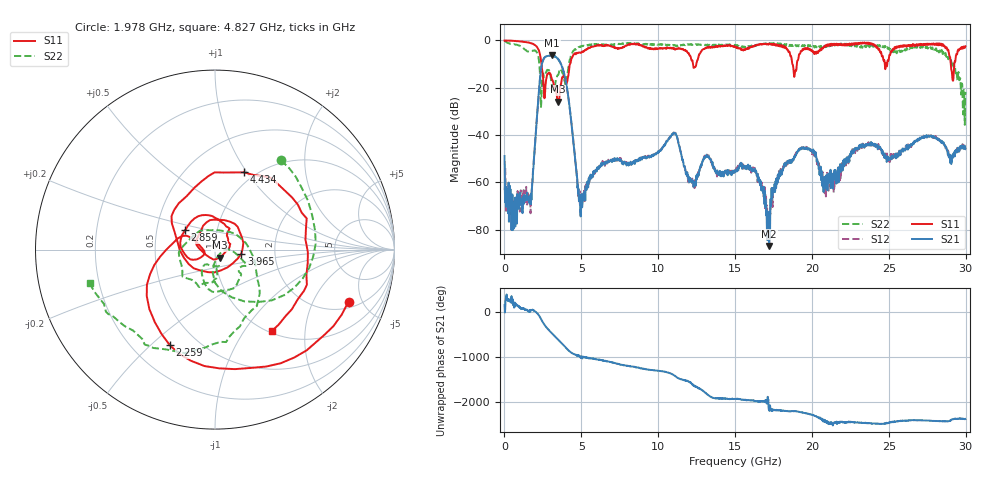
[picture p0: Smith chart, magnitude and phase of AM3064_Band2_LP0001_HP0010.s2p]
# Hz S DB R 50.0
!freq dBS11 angS11 dBS21 angS21 dBS12 angS12 dBS22 angS22
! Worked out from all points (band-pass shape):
!   1600 points, 10 MHz to 29.98 GHz, reference 50 ohm
!   highest |S21| = -6.29 dB at 3.103 GHz (marker M1); lowest = -86.9 dB at 17.22 GHz (marker M2)
!   |S21| within 3 dB of the highest: 2.465 GHz to 3.618 GHz (1.153 GHz wide, 37.9 % of centre)
!   lowest |S11| = -25.9 dB at 3.478 GHz (marker M3), VSWR 1.11, Z = 52.4 - j4.66 ohm
!   |S11| at or under -10 dB: 2.405 GHz to 4.263 GHz (1.858 GHz wide, 55.7 % of centre); 18.73 GHz to 19.02 GHz (291 MHz wide, 1.54 % of centre); 29.03 GHz to 29.26 GHz (229.6 MHz wide, 0.788 % of centre)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
!   |S22| runs from -35.7 to -0.2 dB; largest |S21 - S12| = 0.014
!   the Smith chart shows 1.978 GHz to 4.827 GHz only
!   S11 on the Smith chart (normalised r, x): 1.978 GHz: 2.42, -3.88; 2.259 GHz: 0.35, -0.58; 2.859 GHz: 0.70, +0.16; 3.965 GHz: 1.34, -0.06; 4.434 GHz: 0.89, +0.97; 4.827 GHz: 1.02, -1.35
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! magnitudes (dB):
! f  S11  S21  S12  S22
! 10 MHz  0.0  -48.9  -63.2  -0.2
! 553.6 MHz  -0.2  -68.8  -70.1  -1.6
! 1.603 GHz  -1.0  -67.3  -64.7  -4.7
! 1.978 GHz  -2.0  -44.6  -45.0  -4.2
! 2.259 GHz  -4.6  -19.9  -19.9  -9.6
! 2.859 GHz  -14.0  -6.5  -6.5  -12.6
! 3.103 GHz  -16.9  -6.3  -6.5  -19.3
! 3.478 GHz  -25.9  -7.8  -7.9  -14.6
! 3.965 GHz  -16.5  -16.5  -16.4  -19.1
! 4.434 GHz  -6.7  -39.6  -39.7  -5.0
! 4.827 GHz  -5.1  -65.3  -63.0  -2.8
! 5.015 GHz  -5.1  -65.0  -67.8  -2.6
! 10 GHz  -3.4  -47.5  -46.8  -1.7
! 15 GHz  -2.6  -55.8  -55.3  -1.9
! 16.32 GHz  -2.2  -55.7  -55.2  -2.0
! 17.22 GHz  -1.3  -86.9  -87.0  -1.5
! 17.99 GHz  -2.5  -55.4  -55.2  -1.4
! 19.99 GHz  -4.2  -46.7  -46.8  -2.0
! 20.8 GHz  -2.6  -57.7  -60.0  -2.6
! 25 GHz  -8.1  -50.5  -49.0  -3.1
! 28.56 GHz  -2.2  -43.3  -43.5  -4.9
! 29.98 GHz  -2.5  -45.9  -45.4  -21.8
